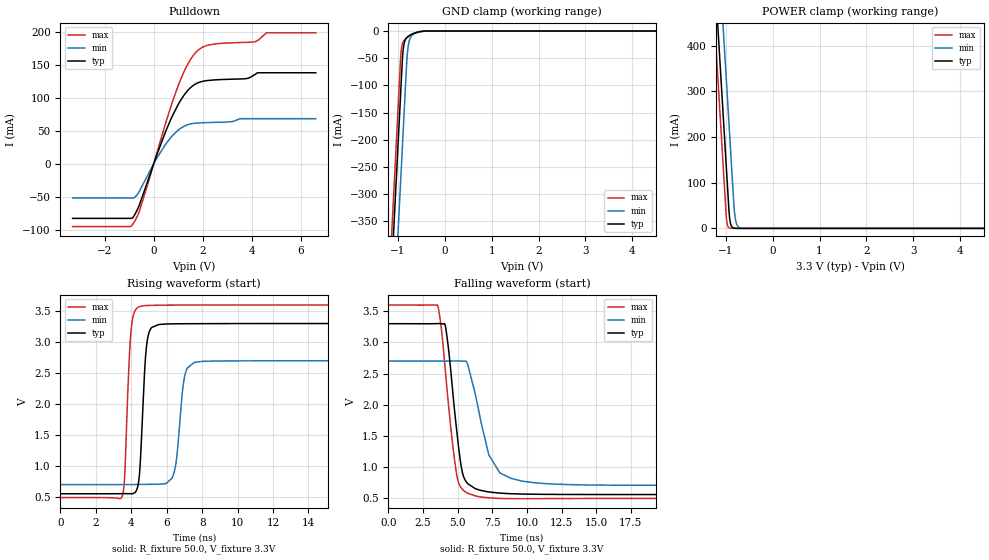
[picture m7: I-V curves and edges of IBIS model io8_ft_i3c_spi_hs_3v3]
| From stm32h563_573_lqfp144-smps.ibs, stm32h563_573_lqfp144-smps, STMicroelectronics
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[Model]   io8_ft_i3c_spi_hs_3v3
Model_type I/O_open_drain
Polarity   Non-Inverting
Enable   Active-Low
| CAP_THRESHOLD on pad IOFT is "UDTCAPC" :
| Rising=20.0% of vddiom   Falling=80.0% of vddiom
| C_comp min and max val. don't necessarily correlate with the min and max pvt
| but are the smallest and greatest pad capacitance found.
| var   typ   min   max
C_comp   3.95813pF  3.95027pF  4.00766pF
|C_comp_pulldown   3.95813pF  3.95027pF  4.00766pF
Vinl = 1.35V
Vinh = 1.8V
Vmeas = 1.65V   | Reference voltage for timing measurements
Cref  = 50.0pF   | Timing specification test load capacitance value
Rref  = 1.0MOhm   | Timing specification test load resistance value
Vref  = 1.815V   | Timing specification test load voltage
[Model Spec]
| TIME_THRESHOLD on pin ZII2CV11 is "CMOS" :
| Rising=40.0% of vdd   Falling=60.0% of vdd
Vinl 1.29880V 1.07480V 1.40680V
Vinh 1.77520V 1.49320V 1.89720V
| variable   typ   min   max
[Temperature Range] 25.0 125.0 -40.0
| variable   typ   min   max
[Voltage Range] 3.3V 2.7V 3.6V
| variable   typ   min   max
[POWER Clamp Reference] 3.3V 2.7V 3.6V
| variable   typ   min   max
[GND Clamp Reference] 0V 0V 0V
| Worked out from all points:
|   slope of the pulldown table from 0 to 0.495 V, typ, clamps not added: 10 ohm
|   GND clamp passes 1 mA (typ) near -0.52 V on its own axis
|   POWER clamp passes 1 mA (typ) near -0.84 V on its own axis
|   rising waveform, R_fixture 50.0, V_fixture 3.3V: 20-80 % time 284ps typ, 381ps min, 266ps max; typ from 0.556 V to 3.3 V
|   falling waveform, R_fixture 50.0, V_fixture 3.3V: 20-80 % time 780ps typ, 1.37ns min, 839ps max; typ from 3.3 V to 0.556 V
[POWER Clamp]
-3.3V     4.068A     4.259A     3.957A
-1.25V    582.8mA    774.2mA    471.5mA
-1.21V    514.8mA    706.2mA    403.5mA
-1.13V    378.8mA    570.2mA    267.5mA
-1.04V    225.8mA    417.2mA    114.5mA
-980mV    123.8mA    315.2mA    17.95mA
-920mV    26.3mA     213.2mA    906uA
-880mV    5.543mA    145.2mA    123.7uA
-810mV    363.5uA    33.6mA     3.798uA
-770mV    76.62uA    10.47mA    519.4nA
-690mV    3.409uA    1.017mA    10.46nA
6.6V      0A         0A         0A
[GND Clamp]
-3.3V     -4.13A     -4.291A    -4.063A
-1.25V    -644.7mA   -806.4mA   -578.1mA
-940mV    -117.7mA   -279.4mA   -51.06mA
-920mV    -83.75mA   -245.4mA   -31.43mA
-900mV    -50.5mA    -211.4mA   -23.14mA
-880mV    -31.27mA   -177.4mA   -19.1mA
-850mV    -18.68mA   -126.4mA   -15.73mA
-800mV    -11.46mA   -46.4mA    -12.03mA
-760mV    -8.752mA   -20.02mA   -9.606mA
-680mV    -5.122mA   -6.673mA   -5.579mA
-300mV    -5.379uA   -47.63uA   -852.7nA
6.6V      10.49nA    1.843uA    393.6pA
| variable   typ   min   max
[Pullup Reference] 3.3V 2.7V 3.6V
| variable   typ   min   max
[Pulldown Reference] 0V 0V 0V
[Pulldown]
-3.3V     -82.42mA   -51.49mA   -94.82mA
-850mV    -81.27mA   -51.49mA   -91.26mA
-580mV    -62.01mA   -41.36mA   -71.41mA
120mV     12.61mA    7.999mA    15.37mA
800mV     75.3mA     43.94mA    97.52mA
1.33V     108.3mA    58.37mA    146.5mA
1.84V     123.1mA    61.83mA    172.7mA
2.51V     126.9mA    62.7mA     181.3mA
3.78V     128.8mA    68.32mA    183.7mA
4.12V     134.9mA    68.32mA    184.6mA
4.59V     137.6mA    68.32mA    198mA
6.6V      137.6mA    68.32mA    198mA
[Ramp]
dV/dt_r 1.64659V/283.08112ps 1.19792V/378.49111ps 1.86382V/262.82881ps
dV/dt_f 1.64666V/779.24086ps 1.19801V/1.25357ns 1.86387V/837.91829ps
R_load = 50.0
| Removed startup time: 0s 0s 0s  .
| Removed end time: 19.4ns.
[Rising Waveform]
R_fixture   = 50.0
V_fixture   = 3.3V
V_fixture_min = 2.7V
V_fixture_max = 3.6V
0s        555.6mV    703.3mV    493.6mV
3.5ns     556.8mV    703.5mV    525.3mV
3.95ns    555.9mV    703.9mV    3.061V
4.4ns     721.1mV    705mV      3.564V
4.8ns     2.751V     706.6mV    3.589V
5.15ns    3.236V     708.2mV    3.593V
6.35ns    3.295V     839.5mV    3.597V
7ns       3.297V     2.435V     3.598V
7.55ns    3.297V     2.674V     3.599V
19.4ns    3.3V       2.7V       3.6V
| Removed startup time: 0s 0s 0s  .
| Removed end time: 39.4ns.
[Falling Waveform]
R_fixture   = 50.0
V_fixture   = 3.3V
V_fixture_min = 2.7V
V_fixture_max = 3.6V
0s        3.3V       2.7V       3.6V
3.55ns    3.302V     2.7V       3.599V
3.85ns    3.3V       2.7V       3.165V
4.15ns    3.218V     2.7V       2.445V
4.9ns     1.647V     2.702V     916.7mV
5.3ns     953.3mV    2.7V       650.1mV
5.75ns    725.9mV    2.627V     574.4mV
7.25ns    596.6mV    1.192V     502.3mV
8.85ns    568.7mV    814.5mV    489.5mV
39.4ns    555.6mV    703.3mV    493.6mV
